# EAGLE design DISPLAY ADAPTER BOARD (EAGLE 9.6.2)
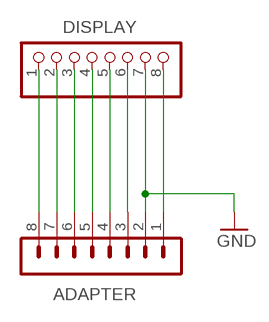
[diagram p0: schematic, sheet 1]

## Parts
ADAPTER  B8B-PH-K-S  [B8B-PH-K-S]
DISPLAY  PINHD-1X8  [1X08]

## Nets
3,3V: ADAPTER.1 DISPLAY.8
BUSY: ADAPTER.8 DISPLAY.1
CS: ADAPTER.5 DISPLAY.4
DC: ADAPTER.6 DISPLAY.3
GND: ADAPTER.2 DISPLAY.7
RES: ADAPTER.7 DISPLAY.2
SCK: ADAPTER.4 DISPLAY.5
SDI: ADAPTER.3 DISPLAY.6

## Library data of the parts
ADAPTER = con-JSTPH:B8B-PH: JST PH series header 2.00mm pitch disconnectable crimp style connectors, vertical (side entry type), 8 pins
DISPLAY = pinhead:PINHD-1X8: PIN HEADER

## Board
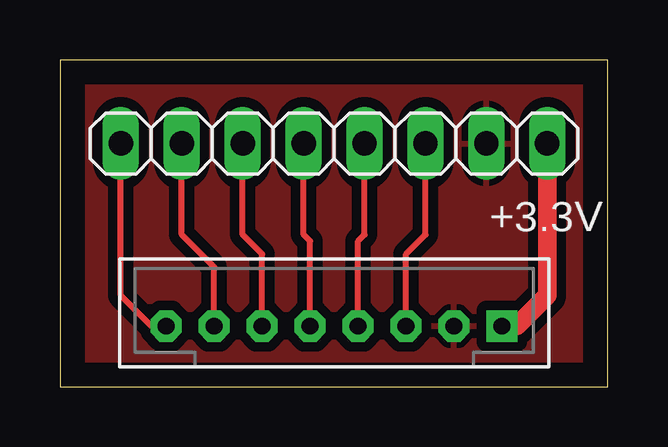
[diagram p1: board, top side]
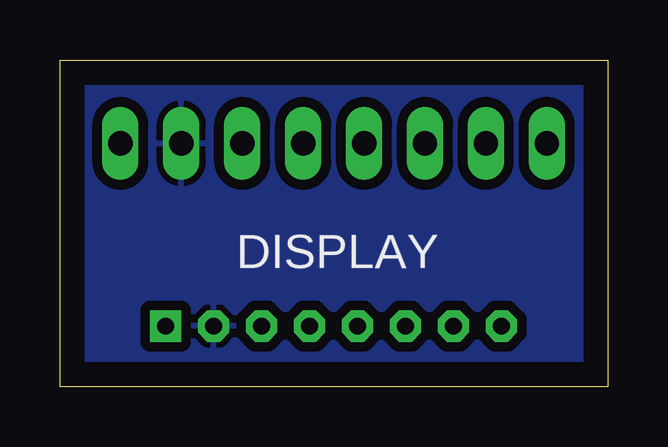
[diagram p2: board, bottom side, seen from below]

Size 22.84 x 13.64 mm. Coordinates in mm from the lower left corner, seen from the top.
Outline: 0,0 22.84,0 22.84,13.64 0,13.64 0,0
Copper layers (1*16): Top 0.035mm / dielectric 1.5mm / Bottom 0.035mm
Design rules "default": minimum track width 6mil, minimum drill 0.35mm, track to track 6mil, track to pad 6mil, pad to pad 6mil, via to via 6mil, smd to smd 6mil, copper to edge 40mil, drill to drill 6mil, minimum pad ring 10mil, minimum via ring 8mil, stop-mask expansion 4mil, vias tented up to drill 0mil, thermal gap 10mil

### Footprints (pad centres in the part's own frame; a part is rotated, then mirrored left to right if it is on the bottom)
B8B-PH-K-S = drill 0.7 pad 1.3 square: 1 7,0 | drill 0.7 pad 1.3 octagon: 2 5,0; 3 3,0; 4 1,0; 5 -1,0; 6 -3,0; 7 -5,0; 8 -7,0
1X08 = drill 1.016 long: 1 -8.89,0; 2 -6.35,0; 3 -3.81,0; 4 -1.27,0; 5 1.27,0; 6 3.81,0; 7 6.35,0; 8 8.89,0

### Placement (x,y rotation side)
ADAPTER  11.43,2.54 0 top
DISPLAY  11.43,10.16 0 top

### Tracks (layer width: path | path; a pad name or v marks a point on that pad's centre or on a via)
3,3V
  Top 0.762: ADAPTER.1 19.05,2.54 20.32,3.81 DISPLAY.8
BUSY
  Top 0.254: ADAPTER.8 3.81,2.54 2.54,3.81 DISPLAY.1
CS
  Top 0.254: DISPLAY.4 10.16,6.35 10.43,6.08 ADAPTER.5
DC
  Top 0.254: ADAPTER.6 8.43,5.54 7.62,6.35 DISPLAY.3
GND
  pour Top (isolate 0.406): 0,13.97 22.86,13.97 22.86,0 0,0
  pour Bottom (isolate 0.406): 0,13.97 22.86,13.97 22.86,0 0,0
RES
  Top 0.254: ADAPTER.7 6.43,5 5.08,6.35 DISPLAY.2
SCK
  Top 0.254: ADAPTER.4 12.43,6.08 12.7,6.35 DISPLAY.5
SDI
  Top 0.254: ADAPTER.3 14.43,5.54 15.24,6.35 DISPLAY.6

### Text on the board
tPlace: +3.3V
bPlace: DISPLAY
